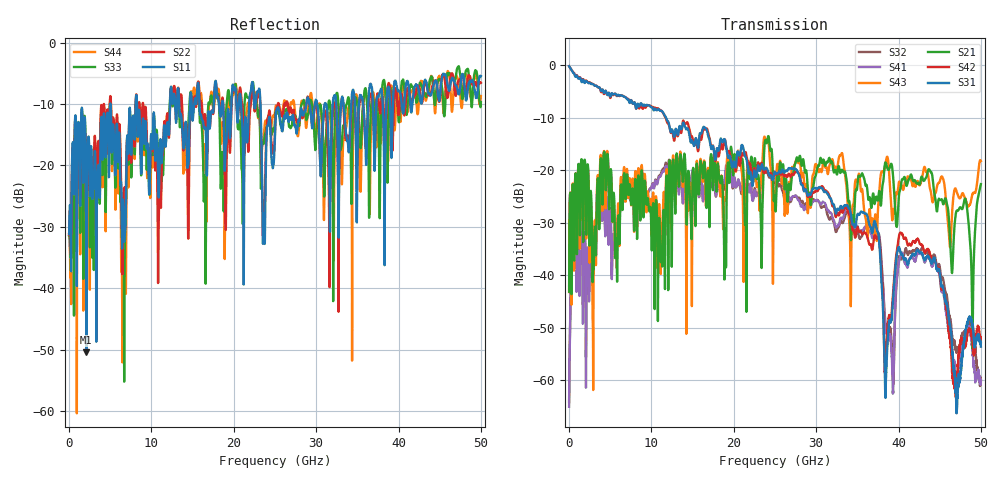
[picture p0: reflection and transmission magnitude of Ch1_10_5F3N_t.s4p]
!Agilent Technologies,N5247A,US51170199,A.09.90.13
!Agilent N5247A: A.09.90.13
!Date: Tuesday, December 08, 2015 12:48:02
!Correction: S11(Full 4 Port(1,2,3,4))
!S12(Full 4 Port(1,2,3,4))
!S13(Full 4 Port(1,2,3,4))
!S14(Full 4 Port(1,2,3,4))
!S21(Full 4 Port(1,2,3,4))
!S22(Full 4 Port(1,2,3,4))
!S23(Full 4 Port(1,2,3,4))
!S24(Full 4 Port(1,2,3,4))
!S31(Full 4 Port(1,2,3,4))
!S32(Full 4 Port(1,2,3,4))
!S33(Full 4 Port(1,2,3,4))
!S34(Full 4 Port(1,2,3,4))
!S41(Full 4 Port(1,2,3,4))
!S42(Full 4 Port(1,2,3,4))
!S43(Full 4 Port(1,2,3,4))
!S44(Full 4 Port(1,2,3,4))
!S4P File: Measurements: <S11,S12,S13,S14>,
!<S21,S22,S23,S24>,
!<S31,S32,S33,S34>,
!<S41,S42,S43,S44>:
# Hz S  dB  R 50
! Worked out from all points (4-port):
!   3201 points, 10 MHz to 50 GHz, reference 50 ohm
!   strongest paths, dB at 10 MHz, 12.51 GHz, 25 GHz, 37.5 GHz, 50 GHz:
!     S31: -0.2, -12.3, -20.4, -31.8, -53.6
!     S42: -0.2, -12.6, -20.4, -32.8, -52.8
!     S21: -43.2, -27.6, -26.1, -25.8, -22.7
!     S43: -43.2, -26.5, -24.4, -27.7, -18.3
!     S41: -65.1, -20.4, -21.9, -31.9, -60.1
!     S32: -64.1, -19.7, -22.5, -32.2, -60.1
!   lowest |S11| = -50.5 dB at 2.103 GHz (marker M1), VSWR 1.01, Z = 49.7 - j0.119 ohm
!   |S11| at or under -10 dB: start of sweep to 5 GHz; 8.248 GHz to 12.26 GHz (4.008 GHz wide, 39.1 % of centre); 23.24 GHz to 28.82 GHz (5.582 GHz wide, 21.4 % of centre)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
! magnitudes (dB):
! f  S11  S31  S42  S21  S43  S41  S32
! 10 MHz  -31.2  -0.2  -0.2  -43.2  -43.2  -65.1  -64.1
! 2.103 GHz  -50.5  -3.0  -3.0  -30.5  -31.0  -41.5  -42.1
! 6.665 GHz  -32.1  -6.0  -6.0  -20.9  -19.5  -25.7  -25.9
! 8.336 GHz  -15.2  -7.4  -7.4  -24.4  -22.7  -23.6  -23.6
! 23.82 GHz  -27.5  -19.7  -20.5  -14.3  -14.0  -20.3  -20.5
! 38.47 GHz  -12.0  -59.7  -54.8  -18.7  -18.4  -50.9  -50.1
! 50 GHz  -5.4  -53.6  -52.8  -22.7  -18.3  -60.1  -60.1
